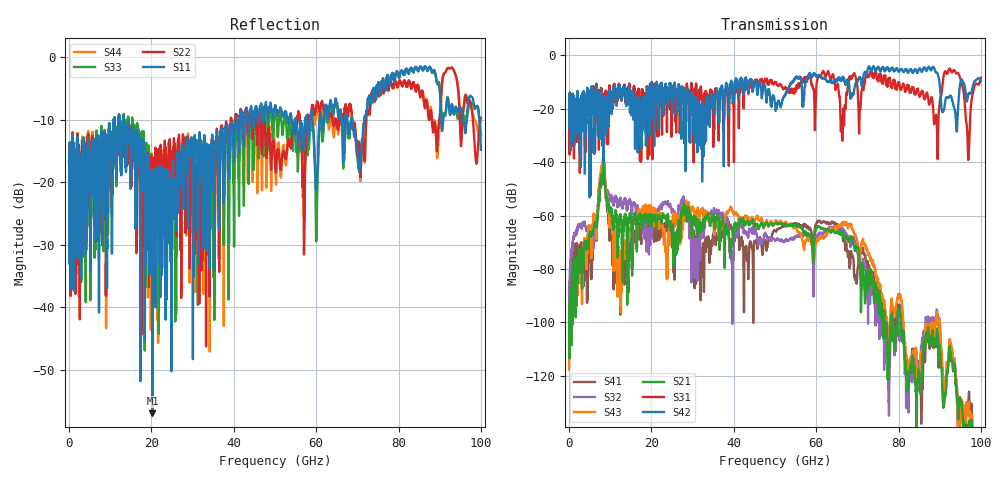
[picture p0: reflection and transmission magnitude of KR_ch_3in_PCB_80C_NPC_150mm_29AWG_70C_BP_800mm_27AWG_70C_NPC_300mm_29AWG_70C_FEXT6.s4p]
# GHz S RI R 45
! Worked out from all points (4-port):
!   4000 points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, 25 MHz to 100 GHz, reference 45 ohm
!   strongest paths, dB at 25 MHz, 25.02 GHz, 50.02 GHz, 75.03 GHz, 100 GHz:
!     S42: -20.7, -17.7, -18.0, -4.4, -9.7
!     S31: -20.7, -15.7, -10.2, -9.4, -8.4
!     S21: -108.6, -69.6, -63.0, -91.0, -168.6
!     S43: -117.6, -62.7, -62.1, -84.2, -163.4
!     S32: -98.5, -58.5, -69.4, -93.9, -179.9
!     S41: -105.1, -68.0, -65.8, -87.9, -162.7
!   lowest |S11| = -56.9 dB at 20.25 GHz (marker M1), VSWR 1.00, Z = 45 - j0.128 ohm
!   |S11| at or under -10 dB: start of sweep to 10.94 GHz; 13.38 GHz to 40.63 GHz (27.26 GHz wide, 101 % of centre); 68.73 GHz to 71.7 GHz (2.972 GHz wide, 4.23 % of centre)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
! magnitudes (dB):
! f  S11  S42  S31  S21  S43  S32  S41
! 25 MHz  -16.5  -20.7  -20.7  -108.6  -117.6  -98.5  -105.1
! 8.1 GHz  -18.9  -22.8  -20.5  -47.5  -42.7  -45.7  -44.4
! 12.3 GHz  -11.0  -12.5  -12.7  -60.2  -81.0  -53.9  -82.0
! 20.25 GHz  -56.9  -12.2  -26.0  -61.5  -59.4  -64.1  -67.6
! 92.5 GHz  -9.2  -15.1  -5.0  -109.8  -106.8  -108.6  -107.8
! 96.88 GHz  -7.6  -15.0  -37.7  -139.1  -134.2  -144.3  -130.2
! 100 GHz  -14.8  -9.7  -8.4  -168.6  -163.4  -179.9  -162.7
